FUNCTION_BLOCK random_dice
VAR_INPUT
	start: BOOL;
	Seed: INT:=500;
	stop: BOOL;

END_VAR

VAR_OUTPUT
	invisible : ARRAY[1..6] OF BOOL;
	visible : ARRAY[1..6] OF STRING;
	buffer : ARRAY [0..65535]OF UINT;
	data: UINT:=1;
	Busy: BOOL;
	Done: BOOL;
END_VAR
VAR
	DRAND1: DRAND;
	Num: LREAL;
	rtirg1:r_TRIG;
	rtirg2: r_TRIG;
	counter: UINT;
	state: INT;
	

	i: INT;
	

END_VAR

(*骰子功能块核心逻辑为，触发功能块之后，使用DRAND功能块产生随机数注意这个功能块需要随机数种子，
同一个程序中使用了多个DRAND时需要设置不同的种子，产生的随机数也不同。
对产生的随机数进行变换和取整，即可得到一个1-6之间的随机数。*)

CASE state OF
	0: 	
		done:=FALSE;	
		FOR i:= 1 TO 6 DO 
			invisible[i]:=TRUE;
		END_FOR
		invisible[1]:=FALSE;
		state:=1;

	1: 
		
		Busy:=FALSE;
		Rtirg1(CLK:= start, Q=> );
		IF Rtirg1.Q THEN
			done:=FALSE;
			Busy:=TRUE;
			state := 2;
		END_IF

	//随机数一直生成	
	2: 
		DRAND1(Seed:= Seed, Num=>Num );    (*Seed随便填，如果一个程序中使用多个DRAND，那么每个Seed就设为不同的数，产生的随机数也会不同*)
		data:=LREAL_TO_UINT(5*Num+1);     (* 产生一个1-6之间的随机整数*)
		rtirg2(CLK:=stop , Q=> );
		// visu_act()这个action是用于配合界面显示使用
		visu_act();
		
	//停止随机数并保存
		IF rtirg2.Q THEN
			Busy:=FALSE;
			done:=TRUE;
			state:=1;
		END_IF



END_CASE

ACTION visu_act:
(*画面中骰子在不同点数之间切换，实际上是给每一个骰子预置了6张图片，
通过切换这些图片的显示与隐藏属性，实现图片之间的切换，达到骰子上的点数在变化的视觉效果*)
CASE data OF 
	0,1: 	invisible[1]	:=	FALSE;
		invisible[2]	:=	TRUE;
		invisible[3]	:=	TRUE;
		invisible[4]	:=	TRUE;
		invisible[5]	:=	TRUE;
		invisible[6]	:=	TRUE;
		
		visible[1]	:=	'Visible';
		visible[2]	:=	'Hidden';
		visible[3]	:=	'Hidden';
		visible[4]	:=	'Hidden';
		visible[5]	:=	'Hidden';
		visible[6]	:=	'Hidden';
		
	2: 	invisible[1]	:=	TRUE;
		invisible[2]	:=	FALSE;
		invisible[3]	:=	TRUE;
		invisible[4]	:=	TRUE;
		invisible[5]	:=	TRUE;
		invisible[6]	:=	TRUE;
		
		
		visible[1]	:=	'Hidden';
		visible[2]	:=	'Visible';
		visible[3]	:=	'Hidden';
		visible[4]	:=	'Hidden';
		visible[5]	:=	'Hidden';
		visible[6]	:=	'Hidden';
		
	3: 	invisible[1]	:=	TRUE;
		invisible[2]	:=	TRUE;
		invisible[3]	:=	FALSE;
		invisible[4]	:=	TRUE;
		invisible[5]	:=	TRUE;
		invisible[6]	:=	TRUE;
		
		
		visible[1]	:=	'Hidden';
		visible[2]	:=	'Hidden';
		visible[3]	:=	'Visible';
		visible[4]	:=	'Hidden';
		visible[5]	:=	'Hidden';
		visible[6]	:=	'Hidden';
		
	4: 	invisible[1]	:=	TRUE;
		invisible[2]	:=	TRUE;
		invisible[3]	:=	TRUE;
		invisible[4]	:=	FALSE;
		invisible[5]	:=	TRUE;
		invisible[6]	:=	TRUE;
		
		visible[1]	:=	'Hidden';
		visible[2]	:=	'Hidden';
		visible[3]	:=	'Hidden';
		visible[4]	:=	'Visible';
		visible[5]	:=	'Hidden';
		visible[6]	:=	'Hidden';
		
	5: 	invisible[1]	:=	TRUE;
		invisible[2]	:=	TRUE;
		invisible[3]	:=	TRUE;
		invisible[4]	:=	TRUE;
		invisible[5]	:=	FALSE;
		invisible[6]	:=	TRUE;
		
		visible[1]	:=	'Hidden';
		visible[2]	:=	'Hidden';
		visible[3]	:=	'Hidden';
		visible[4]	:=	'Hidden';
		visible[5]	:=	'Visible';
		visible[6]	:=	'Hidden';		
		
		
	6: 	invisible[1]	:=	TRUE;
		invisible[2]	:=	TRUE;
		invisible[3]	:=	TRUE;
		invisible[4]	:=	TRUE;
		invisible[5]	:=	TRUE;
		invisible[6]	:=	FALSE;
		
		visible[1]	:=	'Hidden';
		visible[2]	:=	'Hidden';
		visible[3]	:=	'Hidden';
		visible[4]	:=	'Hidden';
		visible[5]	:=	'Hidden';
		visible[6]	:=	'Visible';

END_CASE
END_ACTION

END_FUNCTION_BLOCK
